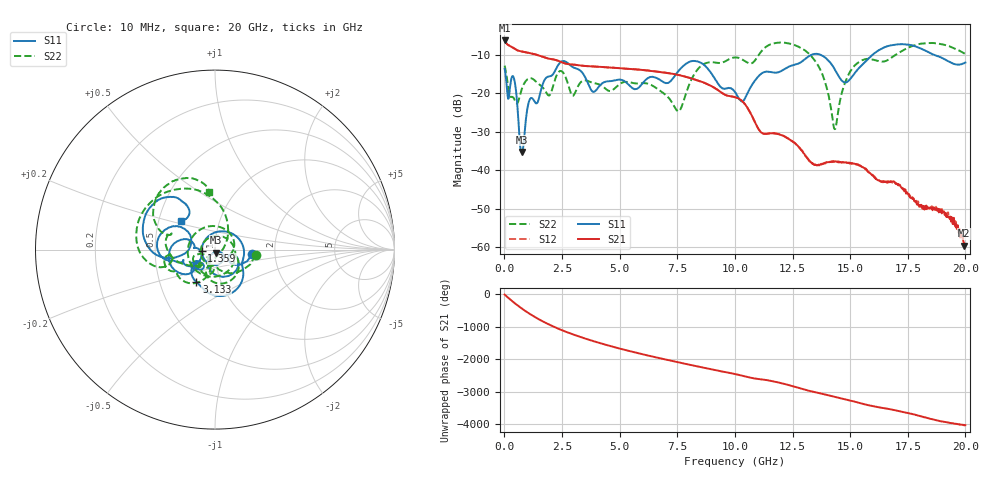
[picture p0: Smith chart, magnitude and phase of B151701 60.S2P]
!  2-Port S-parameters saved by WinCal
! VAR MeasName=S-Parameters (CALIBRATED_DATA) read from VNA (N5244A)
! VAR MeasDate=2015-12-24 19:17:05
! VAR NAME=B151701 60
! VAR FILENAME=B151701 60.S2P
! VAR DATE=2015-12-24 19:17:05
! VAR PHYS_PORTS=1,3
# Hz S DB R 50
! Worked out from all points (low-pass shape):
!   801 points, 10 MHz to 20 GHz, reference 50 ohm
!   highest |S21| = -6.31 dB at 10 MHz (marker M1); lowest = -59.5 dB at 19.95 GHz (marker M2)
!   |S21| within 3 dB of the highest: start of sweep to 878.2 MHz
!   lowest |S11| = -35.2 dB at 759.6 MHz (marker M3), VSWR 1.04, Z = 50.6 - j1.64 ohm
!   |S11| at or under -10 dB: start of sweep to 13.33 GHz; 13.71 GHz to 15.98 GHz (2.273 GHz wide, 15.3 % of centre); 18.63 GHz to end of sweep
!   |S22| runs from -29.3 to -6.8 dB; largest |S21 - S12| = 0.0014
!   S11 on the Smith chart (normalised r, x): 10 MHz: 1.52, -0.07; 1.359 GHz: 0.86, -0.01; 3.133 GHz: 0.76, -0.29; 20 GHz: 0.65, +0.22
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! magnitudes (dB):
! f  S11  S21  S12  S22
! 10 MHz  -13.6  -6.3  -6.3  -12.8
! 434.8 MHz  -16.6  -8.4  -8.4  -21.6
! 759.6 MHz  -35.2  -9.2  -9.2  -18.8
! 1.059 GHz  -22.3  -9.5  -9.5  -16.2
! 1.359 GHz  -22.6  -10.0  -9.9  -16.9
! 1.934 GHz  -15.7  -11.0  -11.0  -20.6
! 2.434 GHz  -12.0  -11.8  -11.8  -14.2
! 3.133 GHz  -13.6  -12.7  -12.7  -19.0
! 3.358 GHz  -14.5  -12.8  -12.8  -16.9
! 3.858 GHz  -19.6  -13.1  -13.0  -17.3
! 6.682 GHz  -16.3  -14.4  -14.4  -19.0
! 7.556 GHz  -14.2  -15.3  -15.2  -24.7
! 8.506 GHz  -12.0  -16.9  -16.9  -13.0
! 10.01 GHz  -19.7  -21.0  -21.0  -10.7
! 12 GHz  -14.2  -30.8  -30.8  -6.8
! 13.35 GHz  -9.9  -38.3  -38.2  -10.6
! 13.88 GHz  -10.6  -38.2  -38.2  -16.4
! 14.33 GHz  -13.8  -37.7  -37.8  -29.3
! 15.13 GHz  -15.3  -38.3  -38.3  -13.3
! 16.68 GHz  -7.7  -42.9  -42.9  -11.2
! 19.95 GHz  -12.2  -59.5  -59.7  -9.7
! 20 GHz  -12.0  -59.3  -58.1  -9.9
